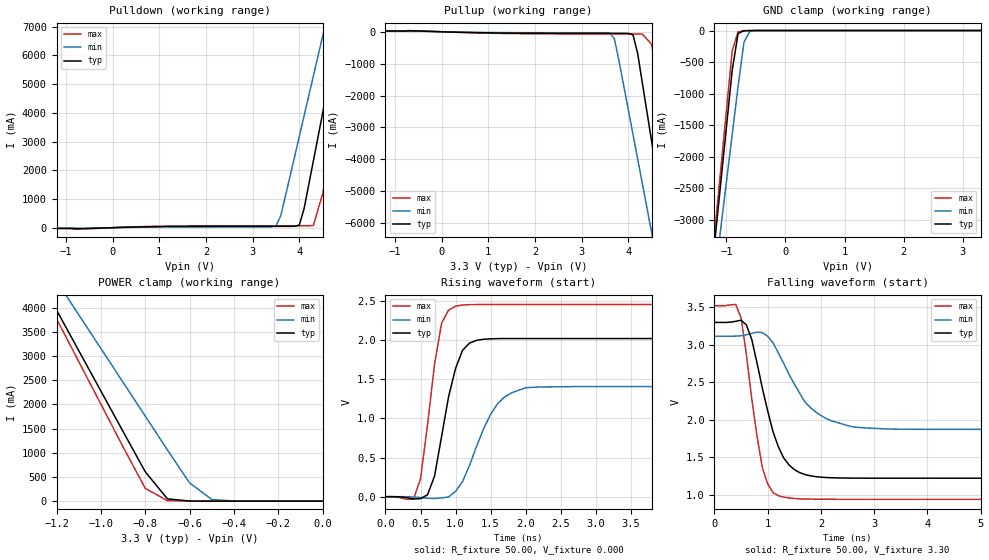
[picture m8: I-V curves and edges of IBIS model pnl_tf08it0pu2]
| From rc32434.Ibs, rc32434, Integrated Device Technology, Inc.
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[Model]   pnl_tf08it0pu2
Model_type   I/O
Polarity   Non-Inverting
Enable   Active-High
Vinl =  0.800V
Vinh =  2.000V
Vmeas =  1.500V
C_comp   0.40pF   0.30pF   0.50pF
[Temperature Range]   25.00   0.12k   0.000
[Voltage Range]   3.30V   3.00V   3.60V
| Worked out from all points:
|   slope of the pulldown table from 0 to 0.495 V, typ, clamps not added: 20.7 ohm
|   slope of the pullup table from 0 to 0.495 V, typ, clamps not added: 24.3 ohm
|   GND clamp passes 1 mA (typ) near -0.62 V on its own axis
|   POWER clamp passes 1 mA (typ) near -0.55 V on its own axis
|   rising waveform, R_fixture 50.00, V_fixture 0.000: 20-80 % time 266ps typ, 412ps min, 214ps max; typ from 0 V to 2.02 V
|   falling waveform, R_fixture 50.00, V_fixture 3.30: 20-80 % time 443ps typ, 655ps min, 305ps max; typ from 3.3 V to 1.22 V
[Pulldown]
| voltage   I(typ)   I(min)   I(max)
-3.3V     -30mA      -30mA      -40mA
3.5V      46.55mA    63.25mA    62.25mA
3.6V      46.66mA    406mA      62.38mA
4V        94.24mA    3.185A     63.29mA
4.1V      655mA      3.883A     64.13mA
4.3V      2.324A     5.281A     74.65mA
4.5V      3.998A     6.679A     1.187A
4.7V      5.672A     8.078A     2.954A
4.9V      7.348A     9.477A     4.721A
5.1V      9.023A     10.87A     6.49A
5.3V      10.7A      12.27A     8.259A
6.6V      21.61A     21.38A     19.78A
[Pullup]
| voltage   I(typ)   I(min)   I(max)
-3.3V     30mA       30mA       40mA
3.6V      -50.04mA   -43.12mA   -68.96mA
3.7V      -50.11mA   -212mA     -69.06mA
3.8V      -50.24mA   -910mA     -69.16mA
4.1V      -96.04mA   -3.218A    -69.76mA
4.2V      -680mA     -3.988A    -71.37mA
4.3V      -1.602A    -4.758A    -75.02mA
4.5V      -3.448A    -6.298A    -393mA
4.7V      -5.294A    -7.839A    -2.332A
4.9V      -7.141A    -9.38A     -4.282A
5.1V      -8.988A    -10.92A    -6.232A
6.6V      -22.85A    -22.48A    -20.87A
[GND_clamp]
| voltage   I(typ)   I(min)   I(max)
-3.3V     -22.79A    -20.13A    -23.71A
-1.2V     -3.397A    -3.957A    -3.237A
-1.1V     -2.474A    -3.187A    -2.262A
-1V       -1.551A    -2.417A    -1.287A
-900mV    -630mA     -1.648A    -323mA
-800mV    -45.7mA    -879mA     -18.37mA
-700mV    -3.145mA   -181mA     -5.441mA
-600mV    -570uA     -12.37mA   -1.875mA
-400mV    -19.37uA   -49.11uA   -48.75uA
3.3V      110pA      101uA      -4.714nA
[POWER_clamp]
| voltage   I(typ)   I(min)   I(max)
-3.3V     21.52A     19.23A     22.31A
-1.3V     4.785A     5.251A     4.652A
-1.2V     3.949A     4.552A     3.769A
-1.1V     3.112A     3.853A     2.886A
-900mV    1.439A     2.456A     1.121A
-800mV    607mA      1.757A     264mA
-700mV    46.95mA    1.059A     10.28mA
-600mV    1.821mA    376mA      1.998mA
-500mV    198uA      33.62mA    614uA
-400mV    23.19uA    1.861mA    90.3uA
0V        110pA      101pA      -715pA
[Ramp]
| variable   typ   min   max
dV/dt_r   1.21/0.27n   0.84/0.41n   1.47/0.21n
dV/dt_f   1.25/0.44n   0.84/0.67n   1.52/0.33n
R_load = 50.00
[Rising Waveform]
R_fixture = 50.00
V_fixture = 0.000
| time   V(typ)   V(min)   V(max)
0s        177uV      145uV      218uV
400ps     -29.49mV   -3.922mV   -28.5mV
500ps     -25.04mV   -10.59mV   227mV
600ps     24.05mV    -19.8mV    917mV
800ps     765mV      -15.26mV   2.214V
1ns       1.638V     68.3mV     2.434V
1.2ns     1.963V     400mV      2.454V
1.6ns     2.02V      1.187V     2.456V
2ns       2.021V     1.392V     2.456V
9.9ns     2.021V     1.407V     2.456V
[Falling Waveform]
R_fixture = 50.00
V_fixture = 3.30
| time   V(typ)   V(min)   V(max)
0s        3.3V       3.115V     3.523V
400ps     3.315V     3.117V     3.539V
500ps     3.329V     3.122V     3.363V
700ps     3.075V     3.153V     2.285V
900ps     2.422V     3.164V     1.361V
1.2ns     1.641V     2.892V     987mV
1.4ns     1.398V     2.607V     957mV
1.8ns     1.252V     2.165V     941mV
2.6ns     1.221V     1.905V     938mV
9.9ns     1.22V      1.872V     938mV
